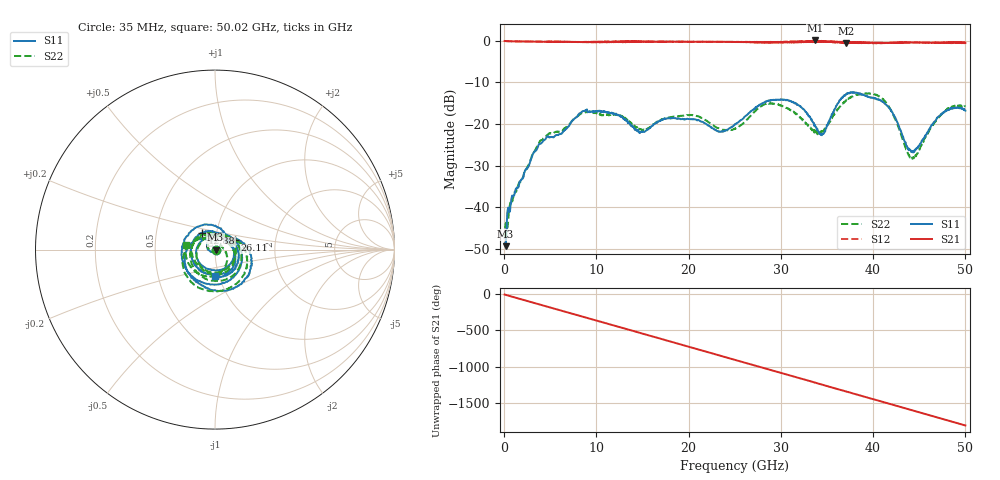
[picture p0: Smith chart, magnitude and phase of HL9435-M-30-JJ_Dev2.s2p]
! 5/26/2020 3:20:00 PM
! H:\PRODUCTION_DATA\TEMP_S2P.S2P
! CHANNEL.1
! TR.MEASUREMENT
! CORRECTED.DATA
# GHZ S RI R 50.0
! FREQ.GHZ  S11RE  S11IM  S21RE  S21IM  S12RE  S12IM  S22RE  S22IM
!; PortSelection: Port_12
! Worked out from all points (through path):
!   1429 points, 35 MHz to 50.02 GHz, reference 50 ohm
!   highest |S21| = 0.09 dB at 33.7 GHz (marker M1); lowest = -0.6 dB at 37.1 GHz (marker M2)
!   group delay of S21, straight-line fit = 101 ps
!   lowest |S11| = -49.4 dB at 140 MHz (marker M3), VSWR 1.01, Z = 50.3 - j0.027 ohm
!   |S11| at or under -10 dB: start of sweep to end of sweep
!   |S22| runs from -47.6 to -12.6 dB; largest |S21 - S12| = 0.045
!   S11 on the Smith chart (normalised r, x): 35 MHz: 1.01, -0.00; 12.88 GHz: 0.85, +0.16; 26.11 GHz: 1.24, +0.13; 50.02 GHz: 0.95, -0.28
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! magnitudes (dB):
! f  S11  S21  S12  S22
! 35 MHz  -48.7  0.0  0.0  -47.6
! 140 MHz  -49.4  -0.1  -0.1  -44.0
! 1.015 GHz  -37.2  -0.1  -0.1  -37.1
! 3.745 GHz  -24.9  -0.2  -0.2  -24.6
! 8.365 GHz  -17.2  -0.3  -0.3  -17.5
! 12.88 GHz  -18.6  -0.4  -0.2  -18.4
! 14.8 GHz  -21.9  -0.1  -0.2  -21.3
! 16.7 GHz  -19.5  -0.2  -0.2  -19.4
! 20.41 GHz  -18.9  -0.2  -0.2  -17.9
! 23.34 GHz  -21.8  -0.2  -0.2  -21.1
! 25.02 GHz  -20.0  -0.2  -0.3  -21.1
! 26.11 GHz  -18.2  -0.3  -0.2  -19.4
! 29.05 GHz  -14.2  -0.3  -0.4  -15.1
! 33.39 GHz  -19.3  -0.1  0.0  -21.5
! 33.7 GHz  -20.2  0.1  -0.2  -21.6
! 34.58 GHz  -22.4  -0.2  -0.2  -21.8
! 37.1 GHz  -12.9  -0.6  -0.3  -14.2
! 39.87 GHz  -13.6  -0.5  -0.6  -12.7
! 41.69 GHz  -16.0  -0.5  -0.5  -15.7
! 44.24 GHz  -26.7  -0.4  -0.4  -28.2
! 47.6 GHz  -17.2  -0.4  -0.5  -17.2
! 50.02 GHz  -16.8  -0.5  -0.5  -15.8
